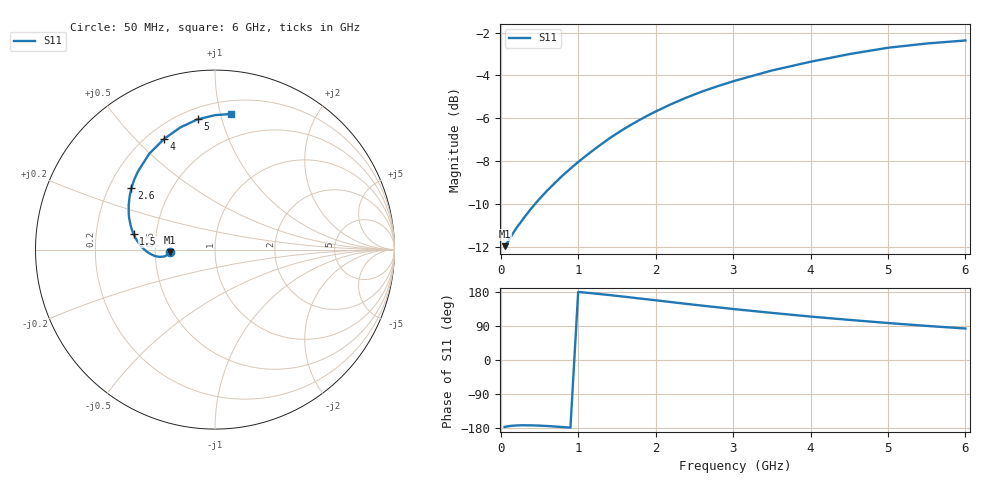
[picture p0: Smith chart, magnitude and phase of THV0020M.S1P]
! SIEMENS Discrete & RF Semiconductors
! BAS70
! Si Schottky Diode in SOT23
! IF = 20 mA
! S-Parameters:  February  1997
# GHz  S  MA  R  50
!  f  S11
! GHz  MAG  ANG
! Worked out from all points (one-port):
!   34 points, 50 MHz to 6 GHz, reference 50 ohm
!   lowest |S11| = -12.0 dB at 50 MHz (marker M1), VSWR 1.67, Z = 29.9 - j0.954 ohm
!   |S11| at or under -10 dB: start of sweep to 443.5 MHz
!   S11 on the Smith chart (normalised r, x): 50 MHz: 0.60, -0.02; 1.5 GHz: 0.37, +0.08; 2.6 GHz: 0.29, +0.30; 4 GHz: 0.27, +0.61; 5 GHz: 0.27, +0.84; 6 GHz: 0.30, +1.08
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0.05  0.2521 -176.6
0.1  0.2594 -174.7
0.15  0.2687 -173.5
0.2  0.2776 -172.8
0.25  0.2853 -172.3
0.4  0.3097 -172.5
0.5  0.325 -173.2
0.6  0.3399 -174.2
0.7  0.3542 -175.5
0.8  0.3686 -177.0
0.9  0.3824 -178.6
1.1  0.4097 177.7
1.3  0.4362 173.6
1.5  0.4619 169.2
1.6  0.4743 166.9
1.8  0.4976 162.2
2  0.5197 157.6
2.2  0.5407 152.8
2.4  0.5603 148.1
2.6  0.5788 143.5
2.8  0.5955 139.1
3  0.6115 134.6
3.5  0.6479 124.4
4  0.6791 114.6
4.5  0.7075 105.9
5  0.7322 97.6
5.5  0.749 90.0
6  0.7614 83.1
